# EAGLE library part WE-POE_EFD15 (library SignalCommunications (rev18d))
Power over Ethernet Transformer Characteristics Flyback transformer designed for PoE PDs Input voltage: 36 V to 57 V Switching frequencies: 200–500 kHz Operating temperature: –40 ºC to +125 ºC Insulation test voltage: 1.5 kVAC/1 min Different output powers and voltages available Applications Suitable for PoE IC’s like LTC4267, TPS 23750, TPS 23770, LM5070, LM 5071, LM 5072 Details see: http://katalog.we-online.de/en/pbs/WE-PoE? Updated by Dan Xu 2014-07-08 2014 (C) Wurth Elektronik
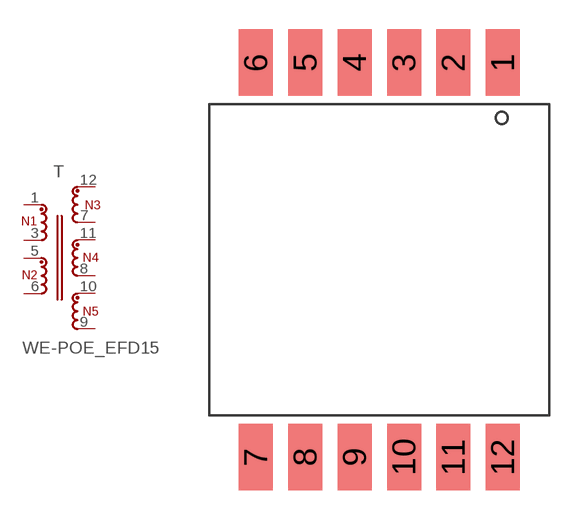
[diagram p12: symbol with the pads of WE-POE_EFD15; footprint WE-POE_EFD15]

Designator prefix T

## WE-POE_EFD15_749119318  [WE-POE_EFD15]
1  1  pas
3  2  pas
5  3  pas
6  4  pas
7  6  pas
8  8  pas
9  10  pas
10  9  pas
11  7  pas
12  5  pas

## WE-POE_EFD15_749119333  [WE-POE_EFD15]
Pads as for WE-POE_EFD15

## WE-POE_EFD15_749119350  [WE-POE_EFD15]
Pads as for WE-POE_EFD15

## Footprint WE-POE_EFD15 (pad centres in mm)
smd 1.75 x 3.43: 1 6.35,10.155; 2 3.81,10.155; 3 1.27,10.155; 4 -1.27,10.155; 5 -3.81,10.155; 6 -6.35,10.155; 7 -6.35,-10.155; 8 -3.81,-10.155; 9 -1.27,-10.155; 10 1.27,-10.155; 11 3.81,-10.155; 12 6.35,-10.155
